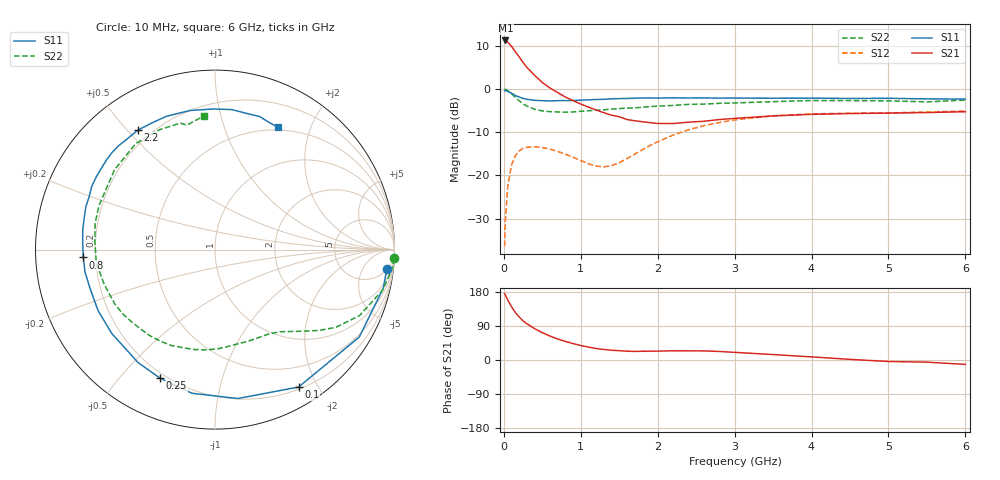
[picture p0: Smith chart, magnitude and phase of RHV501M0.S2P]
! SIEMENS Small Signal Semiconductors
! BFR106
! Si NPN RF Bipolar Junction Transistor in SOT23
! VCE = 0.5 V  IC = 1 mA
! Common Emitter S-Parameters:  August  1996
# GHz  S  MA  R  50
!  f  S11  S21  S12  S22
! GHz  MAG  ANG  MAG  ANG  MAG  ANG  MAG  ANG
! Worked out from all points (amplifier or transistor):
!   36 points, 10 MHz to 6 GHz, reference 50 ohm
!   highest |S21| = 11.3 dB at 20 MHz (marker M1)
!   |S21| within 3 dB of that: start of sweep to 166.1 MHz
!   unconditionally stable (mu >= 1): 799.4 MHz to end of sweep
!   at 250 MHz: K = 0.33, MSG = 10.0 dB, |S12| = -13.7 dB
!   at 1.4 GHz: K = 1.65, MAG = 1.1 dB, |S12| = -17.7 dB
!   at 6 GHz: K = 1.02, MAG = -1.0 dB, |S12| = -5.1 dB
!   S11 on the Smith chart (normalised r, x): 10 MHz: 6, -16; 100 MHz: 0.23, -1.76; 250 MHz: 0.18, -0.64; 800 MHz: 0.15, -0.03; 2.2 GHz: 0.15, +0.54; 6 GHz: 0.47, +1.54
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0.01  0.9634 -6.3  3.648 175.1  0.0152 87.0  0.9986 -2.8
0.02  0.9622 -12.8  3.654 171.5  0.0305 81.5  0.9957 -5.6
0.05  0.94 -31.2  3.496 158.4  0.074 71.3  0.9622 -13.4
0.1  0.8962 -58.7  3.125 140.8  0.1327 55.8  0.8855 -24.5
0.15  0.8394 -81.3  2.705 124.9  0.1694 43.0  0.8001 -32.8
0.2  0.8106 -99.1  2.354 113.5  0.1925 34.1  0.7319 -38.0
0.25  0.7787 -113.2  2.032 103.2  0.2055 26.7  0.6725 -42.5
0.3  0.7616 -124.2  1.785 95.6  0.2119 21.6  0.6356 -45.8
0.4  0.7411 -141.1  1.44 82.8  0.2149 13.2  0.584 -51.6
0.5  0.7346 -152.5  1.193 72.2  0.2107 7.6  0.5582 -57.2
0.6  0.7289 -162.3  1.029 63.2  0.2018 3.8  0.5474 -63.2
0.8  0.7352 -176.6  0.809 49.1  0.1763 0.6  0.5402 -75.8
1.1  0.7502 166.2  0.618 34.0  0.1365 7.8  0.5612 -95.3
1.4  0.7713 152.9  0.499 25.8  0.1298 31.3  0.5876 -114.7
1.9  0.7896 132.8  0.409 23.3  0.222 51.6  0.6274 -145.6
2.2  0.7923 122.7  0.399 24.3  0.2935 49.2  0.6468 -162.6
2.8  0.7861 105.0  0.444 22.5  0.4099 36.7  0.6837 167.7
3.5  0.7836 90.6  0.489 14.3  0.4902 21.6  0.7152 141.5
4.5  0.7788 76.8  0.521 1.7  0.5252 4.6  0.7363 114.9
5  0.7821 71.5  0.527 -4.0  0.5291 -1.5  0.7306 105.3
5.5  0.7698 66.7  0.535 -5.7  0.5433 -4.4  0.7111 102.8
6  0.7665 62.8  0.547 -11.6  0.5569 -10.9  0.7471 94.7
